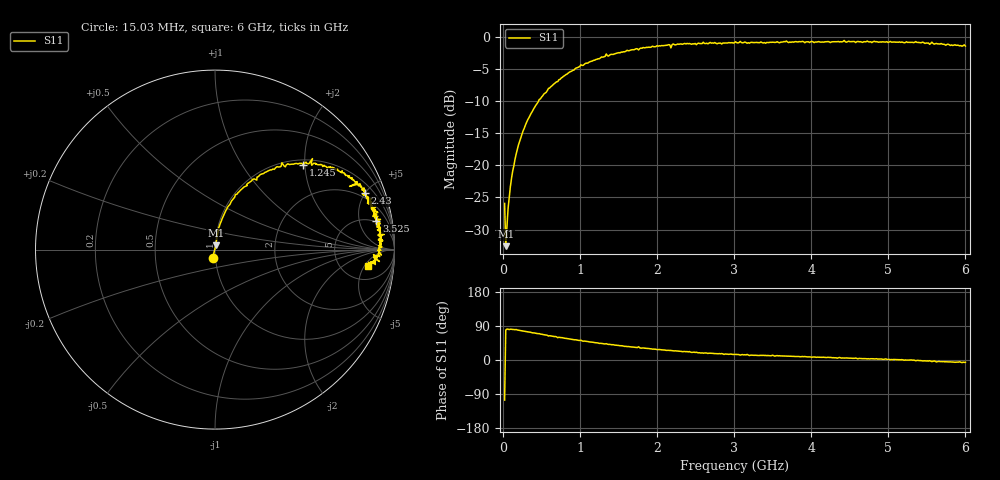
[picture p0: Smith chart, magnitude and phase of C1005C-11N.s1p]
!	Network	Analyzer	HP8753E.07.74:	Oct	30	2002	Serial	No.	JP38451487
!	Hewlett-Packard
!	7	Sep	2009	8:41:45
!	Frequency	S11
#	HZ	S	RI	R	50
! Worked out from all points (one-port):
!   400 points, 15.03 MHz to 6 GHz, reference 50 ohm
!   lowest |S11| = -32.6 dB at 30.03 MHz (marker M1), VSWR 1.05, Z = 50.4 + j2.32 ohm
!   |S11| at or under -10 dB: start of sweep to 453.5 MHz
!   S11 on the Smith chart (normalised r, x): 15.03 MHz: 0.97, -0.09; 1.245 GHz: 1.12, +1.96; 2.43 GHz: 1.61, +4.95; 3.525 GHz: 5, +9; 6 GHz: 9, -6
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1.502992e7  -0.0138 -0.0486
3.002985e7  0.00448 0.023
6.00297e7  0.00692 0.0456
1.050295e8  0.0125 0.0785
1.650292e8  0.0203 0.121
2.400288e8  0.0394 0.171
4.650277e8  0.114 0.307
7.650262e8  0.252 0.418
1.005025e9  0.373 0.484
1.245024e9  0.492 0.471
1.335023e9  0.543 0.507
1.515022e9  0.6 0.463
1.99502e9  0.764 0.398
2.160019e9  0.792 0.372
2.175019e9  0.75 0.352
2.205019e9  0.81 0.365
2.265019e9  0.813 0.357
2.430018e9  0.833 0.316
3.015015e9  0.894 0.236
3.195014e9  0.882 0.184
3.495013e9  0.895 0.201
3.525012e9  0.899 0.161
3.765011e9  0.905 0.158
4.515007e9  0.924 0.0787
5.265004e9  0.916 -0.0025
5.595002e9  0.885 -0.0403
5.625002e9  0.893 -0.0831
6e9  0.851 -0.0915
